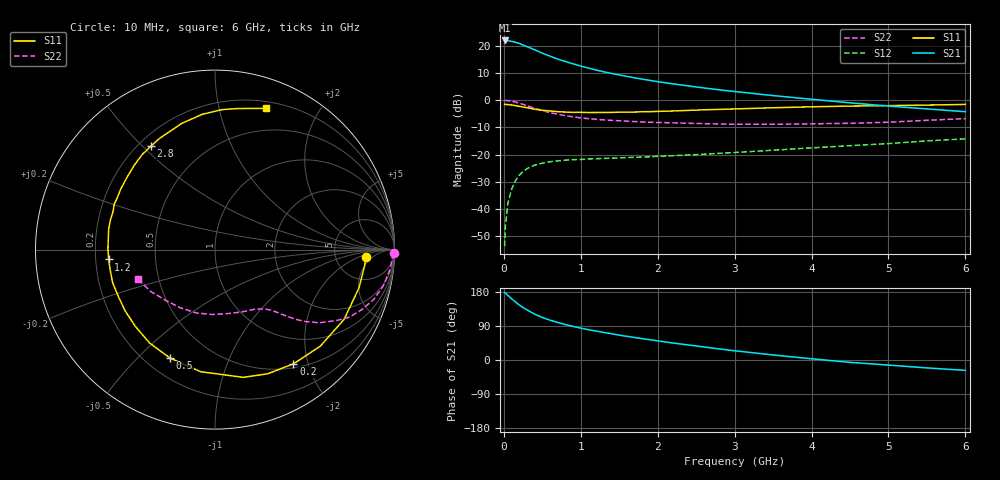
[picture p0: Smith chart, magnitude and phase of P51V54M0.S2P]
! SIEMENS Small Signal Semiconductors
! BFP183
! Si NPN RF Bipolar Junction Transistor in SOT143
! VCE = 1.5 V  IC = 4 mA
! Common Emitter S-Parameters:  March  1996
# GHz  S  MA  R  50
!  f  S11  S21  S12  S22
! GHz  MAG  ANG  MAG  ANG  MAG  ANG  MAG  ANG
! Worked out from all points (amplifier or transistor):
!   36 points, 10 MHz to 6 GHz, reference 50 ohm
!   highest |S21| = 21.9 dB at 10 MHz (marker M1)
!   |S21| within 3 dB of that: start of sweep to 365 MHz
!   unconditionally stable (mu >= 1): 1.648 GHz to 5.806 GHz
!   at 250 MHz: K = 0.18, MSG = 23.2 dB, |S12| = -26.1 dB
!   at 1.4 GHz: K = 0.89, MSG = 15.5 dB, |S12| = -21.2 dB
!   at 6 GHz: K = 0.97, MSG = 5.0 dB, |S12| = -14.2 dB
!   S11 on the Smith chart (normalised r, x): 10 MHz: 11, -3; 200 MHz: 0.56, -1.76; 500 MHz: 0.30, -0.63; 1.2 GHz: 0.25, -0.04; 2.8 GHz: 0.25, +0.53; 6 GHz: 0.27, +1.39
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0.01  0.8411 -2.9  12.49 178.4  0.0021 88.0  0.9948 -1.2
0.02  0.8386 -6.1  12.44 176.9  0.0047 85.0  0.9889 -2.5
0.05  0.8302 -14.9  12.46 170.8  0.0124 81.6  0.9829 -6.1
0.1  0.8175 -28.4  12.02 161.9  0.023 74.8  0.9597 -12.1
0.15  0.7959 -42.6  11.54 153.3  0.0332 67.5  0.9263 -17.5
0.2  0.7721 -55.5  11.03 145.3  0.0423 62.1  0.8831 -22.3
0.25  0.7516 -67.0  10.27 138.4  0.0493 56.2  0.8389 -26.6
0.3  0.729 -77.5  9.65 132.4  0.0554 52.1  0.7928 -29.7
0.4  0.6851 -96.7  8.431 121.0  0.0644 44.2  0.7125 -34.9
0.5  0.6542 -112.5  7.295 112.1  0.0699 38.4  0.644 -38.5
0.6  0.6356 -124.9  6.449 105.2  0.0743 34.7  0.5927 -40.9
0.7  0.6167 -135.8  5.676 99.0  0.0773 32.0  0.5525 -42.5
0.8  0.6061 -145.7  5.13 93.5  0.0795 29.4  0.5215 -43.9
1.1  0.5948 -169.0  3.892 79.9  0.0837 25.7  0.4588 -47.3
1.2  0.5953 -174.7  3.582 76.3  0.0845 24.7  0.4467 -48.5
1.7  0.6061 159.7  2.577 59.4  0.0897 24.2  0.4062 -54.9
2.2  0.6346 140.5  1.995 44.8  0.096 25.0  0.3844 -63.0
2.8  0.6779 121.9  1.553 29.2  0.1061 26.3  0.3664 -75.3
3.5  0.7268 104.9  1.216 13.3  0.121 26.6  0.3618 -92.2
4.5  0.7807 87.2  0.896 -6.2  0.1467 24.1  0.3776 -121.1
5.5  0.8143 75.0  0.693 -20.9  0.1797 20.0  0.4284 -147.2
6  0.8366 70.0  0.615 -27.4  0.1951 16.1  0.4599 -159.3
